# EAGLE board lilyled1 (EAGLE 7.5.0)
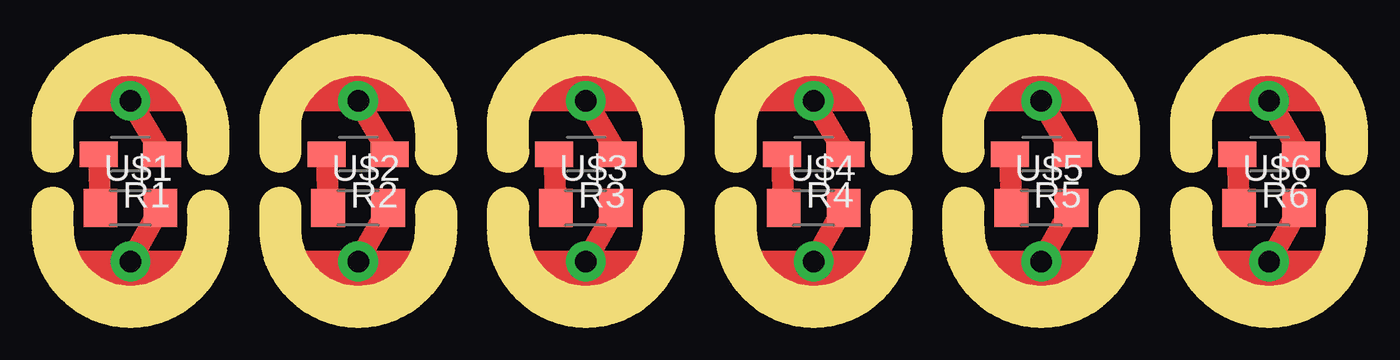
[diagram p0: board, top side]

Size 61.34 x 11.96 mm. Coordinates in mm from the lower left corner, seen from the top.
Outline: 7.37,7.24 7.37,8.38 arc166 0,9.02 0,7.37
Outline: 7.37,4.57 7.37,3.68 arc-180 0,3.68 0,4.7
Outline: 18.16,7.24 18.16,8.38 arc166 10.79,9.02 10.79,7.37
Outline: 18.16,4.57 18.16,3.68 arc-180 10.79,3.68 10.79,4.7
Outline: 28.96,7.24 28.96,8.38 arc166 21.59,9.02 21.59,7.37
Outline: 28.96,4.57 28.96,3.68 arc-180 21.59,3.68 21.59,4.7
Outline: 39.75,7.24 39.75,8.38 arc166 32.38,9.02 32.38,7.37
Outline: 39.75,4.57 39.75,3.68 arc-180 32.38,3.68 32.38,4.7
Outline: 50.55,7.24 50.55,8.38 arc166 43.18,9.02 43.18,7.37
Outline: 50.55,4.57 50.55,3.68 arc-180 43.18,3.68 43.18,4.7
Outline: 61.34,7.24 61.34,8.38 arc166 53.97,9.02 53.97,7.37
Outline: 61.34,4.57 61.34,3.68 arc-180 53.97,3.68 53.97,4.7
Copper layers (1*16): Top 0.035mm / dielectric 1.5mm / Bottom 0.035mm
Design rules "default": minimum track width 10mil, minimum drill 24mil, track to track 8mil, track to pad 8mil, pad to pad 8mil, via to via 8mil, smd to smd 8mil, copper to edge 40mil, drill to drill 8mil, minimum pad ring 10mil, minimum via ring 8mil, stop-mask expansion 4mil, vias tented up to drill 0mil, thermal gap 10mil

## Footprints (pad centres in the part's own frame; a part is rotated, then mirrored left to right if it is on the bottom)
1X01NS-KIT = drill 1.016 pad 1.88: 1 0,0
R1206W = smd 1.8 x 1.2: 1 -1.499,0; 2 1.499,0
LED1206 = smd 1.6 x 1.803: 1 -1.422,0; 2 1.422,0

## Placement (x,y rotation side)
J1  [1X01NS-KIT]  3.68,9.78 0 top
J2  [1X01NS-KIT]  3.68,2.16 0 top
J3  [1X01NS-KIT]  14.48,9.78 0 top
J4  [1X01NS-KIT]  14.48,2.16 0 top
J5  [1X01NS-KIT]  25.27,9.78 0 top
J6  [1X01NS-KIT]  25.27,2.16 0 top
J7  [1X01NS-KIT]  36.07,9.78 0 top
J8  [1X01NS-KIT]  36.07,2.16 0 top
J9  [1X01NS-KIT]  46.86,9.78 0 top
J10  [1X01NS-KIT]  46.86,2.16 0 top
J11  [1X01NS-KIT]  57.66,9.78 0 top
J12  [1X01NS-KIT]  57.66,2.16 0 top
R1  [R1206W]  3.68,7.24 180 top
R2  [R1206W]  14.48,7.24 180 top
R3  [R1206W]  25.27,7.24 180 top
R4  [R1206W]  36.07,7.24 180 top
R5  [R1206W]  46.86,7.24 180 top
R6  [R1206W]  57.66,7.24 180 top
U$1  LED  [LED1206]  3.68,4.7 0 top
U$2  LED  [LED1206]  14.48,4.7 0 top
U$3  LED  [LED1206]  25.27,4.7 0 top
U$4  LED  [LED1206]  36.07,4.7 0 top
U$5  LED  [LED1206]  46.86,4.7 0 top
U$6  LED  [LED1206]  57.66,4.7 0 top

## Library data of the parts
J1-J12 = SparkFun-Connectors
R1-R6 U$1-U$6 = fab

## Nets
GND: J2.1 U$1.2
GND1: J4.1 U$2.2
GND2: J6.1 U$3.2
GND3: J8.1 U$4.2
GND4: J10.1 U$5.2
GND5: J12.1 U$6.2
N$1: R1.2 U$1.1
N$2: R2.2 U$2.1
N$3: R3.2 U$3.1
N$4: R4.2 U$4.1
N$5: R5.2 U$5.1
N$6: R6.2 U$6.1
VCC: J1.1 R1.1
VCC1: J3.1 R2.1
VCC2: J5.1 R3.1
VCC3: J7.1 R4.1
VCC4: J9.1 R5.1
VCC5: J11.1 R6.1

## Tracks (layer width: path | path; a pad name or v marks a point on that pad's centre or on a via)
GND
  Top 1.016: J2.1 U$1.2 | J2.1 1.78,2.16 | J2.1 5.59,2.16 | 5.59,2.16 4.95,1.52 2.41,1.52 | 5.59,2.16 6.22,2.16 | 5.59,2.16 1.14,2.16
GND1
  Top 1.016: J4.1 U$2.2 | J4.1 12.57,2.16 | J4.1 16.38,2.16 | 16.38,2.16 15.75,1.52 13.21,1.52 | 16.38,2.16 17.02,2.16 | 16.38,2.16 11.94,2.16
GND2
  Top 1.016: J6.1 U$3.2 | J6.1 23.37,2.16 | J6.1 27.18,2.16 | 27.18,2.16 26.54,1.52 24,1.52 | 27.18,2.16 27.81,2.16 | 27.18,2.16 22.73,2.16
GND3
  Top 1.016: J8.1 U$4.2 | J8.1 34.16,2.16 | J8.1 37.97,2.16 | 37.97,2.16 37.34,1.52 34.8,1.52 | 37.97,2.16 38.61,2.16 | 37.97,2.16 33.53,2.16
GND4
  Top 1.016: J10.1 U$5.2 | J10.1 44.96,2.16 | J10.1 48.77,2.16 | 48.77,2.16 48.13,1.52 45.59,1.52 | 48.77,2.16 49.4,2.16 | 48.77,2.16 44.32,2.16
GND5
  Top 1.016: J12.1 U$6.2 | J12.1 55.75,2.16 | J12.1 59.56,2.16 | 59.56,2.16 58.93,1.52 56.39,1.52 | 59.56,2.16 60.2,2.16 | 59.56,2.16 55.12,2.16
N$1
  Top 1.016: R1.2 U$1.1
N$2
  Top 1.016: R2.2 U$2.1
N$3
  Top 1.016: R3.2 U$3.1
N$4
  Top 1.016: R4.2 U$4.1
N$5
  Top 1.016: R5.2 U$5.1
N$6
  Top 1.016: R6.2 U$6.1
VCC
  Top 1.016: J1.1 R1.1 | J1.1 5.59,9.78 | J1.1 1.78,9.78 | 1.78,9.78 3.05,10.41 3.68,10.41 3.68,11.05 4.32,10.41 5.59,10.41 3.05,11.05 2.41,10.41 1.78,10.41 | 1.78,9.78 1.14,9.78 | 1.78,9.78 6.22,9.78
VCC1
  Top 1.016: J3.1 R2.1 | J3.1 16.38,9.78 | J3.1 12.57,9.78 | 12.57,9.78 13.84,10.41 14.48,10.41 14.48,11.05 15.11,10.41 16.38,10.41 13.84,11.05 13.21,10.41 12.57,10.41 | 12.57,9.78 11.94,9.78 | 12.57,9.78 17.02,9.78
VCC2
  Top 1.016: J5.1 R3.1 | J5.1 27.18,9.78 | J5.1 23.37,9.78 | 23.37,9.78 24.64,10.41 25.27,10.41 25.27,11.05 25.91,10.41 27.18,10.41 24.64,11.05 24,10.41 23.37,10.41 | 23.37,9.78 22.73,9.78 | 23.37,9.78 27.81,9.78
VCC3
  Top 1.016: J7.1 R4.1 | J7.1 37.97,9.78 | J7.1 34.16,9.78 | 34.16,9.78 35.43,10.41 36.07,10.41 36.07,11.05 36.7,10.41 37.97,10.41 35.43,11.05 34.8,10.41 34.16,10.41 | 34.16,9.78 33.53,9.78 | 34.16,9.78 38.61,9.78
VCC4
  Top 1.016: J9.1 R5.1 | J9.1 48.77,9.78 | J9.1 44.96,9.78 | 44.96,9.78 46.23,10.41 46.86,10.41 46.86,11.05 47.5,10.41 48.77,10.41 46.23,11.05 45.59,10.41 44.96,10.41 | 44.96,9.78 44.32,9.78 | 44.96,9.78 49.4,9.78
VCC5
  Top 1.016: J11.1 R6.1 | J11.1 59.56,9.78 | J11.1 55.75,9.78 | 55.75,9.78 57.02,10.41 57.66,10.41 57.66,11.05 58.29,10.41 59.56,10.41 57.02,11.05 56.39,10.41 55.75,10.41 | 55.75,9.78 55.12,9.78 | 55.75,9.78 60.2,9.78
